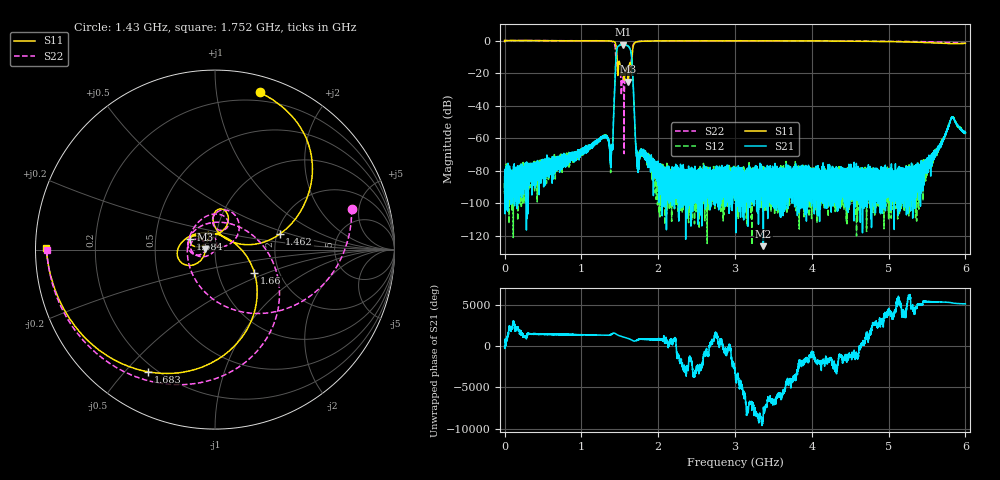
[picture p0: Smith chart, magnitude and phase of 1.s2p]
!Keysight Technologies,N5232A,MY52221221,A.10.65.11
!Date: Wednesday, January 10, 2024 14:27:23
!Correction: S11(Full 2 Port(1,4))
!S41(Full 2 Port(1,4))
!S14(Full 2 Port(1,4))
!S44(Full 2 Port(1,4))
!S2P File: Measurements: S11, S41, S14, S44:
# Hz S  RI  R 50
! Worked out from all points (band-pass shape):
!   16001 points, 300 kHz to 6 GHz, reference 50 ohm
!   highest |S21| = -2.44 dB at 1.54 GHz (marker M1); lowest = -126.3 dB at 3.369 GHz (marker M2)
!   |S21| within 3 dB of the highest: 1.462 GHz to 1.636 GHz (173.5 MHz wide, 11.2 % of centre)
!   lowest |S11| = -25.4 dB at 1.608 GHz (marker M3), VSWR 1.11, Z = 44.9 + j0.233 ohm
!   |S11| at or under -10 dB: 1.464 GHz to 1.661 GHz (197.6 MHz wide, 12.6 % of centre)
!   |S22| runs from -69.5 to 0.0 dB; largest |S21 - S12| = 0.0071
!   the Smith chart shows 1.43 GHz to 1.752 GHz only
!   S11 on the Smith chart (normalised r, x): 1.43 GHz: 0.13, +1.31; 1.462 GHz: 2.07, +0.41; 1.584 GHz: 0.75, +0.09; 1.66 GHz: 1.49, -0.41; 1.683 GHz: 0.17, -0.58; 1.752 GHz: 0.03, +0.00
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300000  1.004 -0.00833  6.41e-05 -1.09e-05  -6.79e-06 -4.15e-05  1.003 -0.00961
4.679016e8  0.00429 -0.9946  0.000169 8.71e-06  8.78e-05 5.36e-05  0.0341 -0.9925
1.000375e9  -0.9711 -0.1374  0.000174 -0.00033  0.000178 -0.000347  -0.98 -0.0579
1.382481e9  -0.3242 0.9092  5.51e-05 -0.000109  2.07e-07 -0.000125  0.1082 0.9449
1.430478e9  0.2481 0.8758  -0.0144 0.0217  -0.0138 0.0217  0.7614 0.2262
1.461977e9  0.3602 0.0859  0.4018 -0.3428  0.4063 -0.3419  0.0428 0.1904
1.50135e9  0.0745 0.1763  -0.6598 0.2922  -0.6602 0.2971  0.1348 0.1169
1.539598e9  -0.0357 0.0936  0.5278 0.5403  0.5305 0.5382  -0.0105 0.0697
1.583846e9  -0.1394 0.0607  0.1899 -0.6913  0.1902 -0.695  -0.1366 0.0205
1.607845e9  -0.0538 0.00259  -0.5695 -0.3692  -0.574 -0.3672  -0.0539 0.01
1.659592e9  0.2193 -0.1291  0.199 -0.0845  0.1986 -0.0874  0.3546 -0.3132
1.682841e9  -0.3716 -0.6811  -0.0064 -0.0147  -0.00617 -0.0147  -0.333 -0.7392
1.718839e9  -0.8657 -0.2851  0.000319 -0.000233  0.00035 -0.00018  -0.8523 -0.3297
1.751837e9  -0.9397 0.00881  -3.51e-05 0.000282  -7.17e-05 0.000241  -0.9379 -0.00241
2.00045e9  -0.5821 0.7796  -6.02e-06 0.00015  5.68e-05 0.000135  -0.4531 0.8569
3.00015e9  0.811 0.5428  2.34e-05 -2.72e-05  3.79e-05 9.76e-05  0.9548 0.1928
3.369132e9  0.9758 0.0808  3.01e-07 3.77e-07  -1.75e-05 -6.17e-06  0.9126 -0.3459
4.000225e9  0.6837 -0.6939  -7.27e-06 2.01e-05  6.81e-06 -1.64e-05  0.2897 -0.9245
5.0003e9  -0.6829 -0.6312  8.05e-05 3.72e-05  -8.29e-06 -6.56e-05  -0.8547 -0.4038
5.684641e9  -0.2188 0.7994  0.00024 -0.00062  0.000263 -0.000754  -0.4986 0.7319
5.827134e9  0.333 0.7304  -0.0044 -0.000475  -0.00438 -0.000415  -0.1194 0.8519
6e9  0.8011 0.1885  0.000478 0.0014  0.000488 0.00143  0.4423 0.6961
